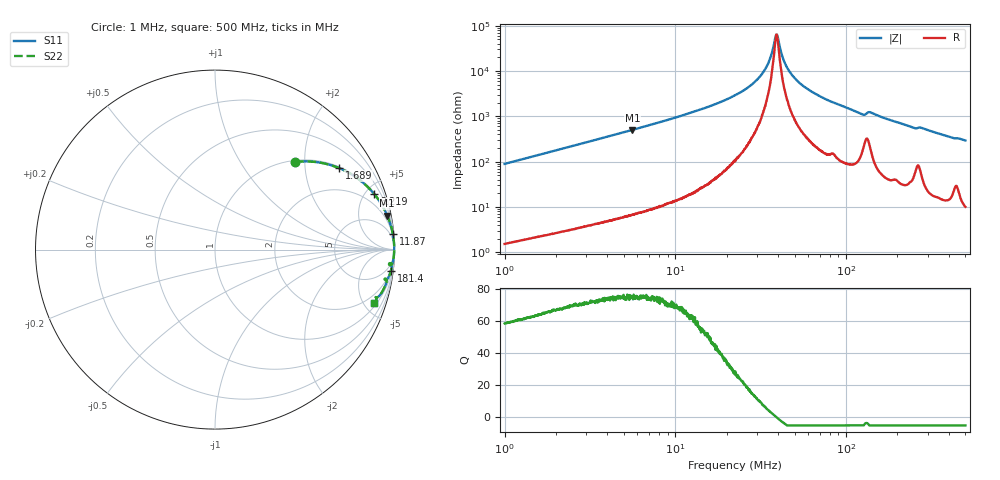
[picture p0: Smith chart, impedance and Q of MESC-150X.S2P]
!s-Parameter Generated by FASTRON Sdn. Bhd.
!FASTRON P/N : MESC-150X
!Keysight Technologies,E4991B,MY54100416,A.01.15
!Date: Mon Mar 16 10:57:22 2026
!Version  : Rev00 Mon Mar 16 10:57:22 2026
!Data & Calibration Information:
!PortZ  Port1:50+j0  Port2:50+j0
!When reading, reference impedance value at option line is always used.
!Remarks : This data is being provided solely for informational purposes.
!Freq	S11	S21	S12	S22
# Hz S dB R 50
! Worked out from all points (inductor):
!   1601 points, 1 MHz to 500 MHz, reference 50 ohm
!   read as one part in series: L = 14.2 uH near 1.032 MHz
!   highest Q = 75.5 at 5.61 MHz (marker M1), where L = 14.3 uH
!   self-resonance near 39.12 MHz
!   S11 on the Smith chart (normalised r, x): 1 MHz: 1.03, +1.79; 1.689 MHz: 1.05, +3.01; 3.219 MHz: 1.08, +5.73; 11.87 MHz: 1, +23; 181.4 MHz: 2, -17; 500 MHz: 1.20, -5.88
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1000000  -3.59 47.6  -2.63 -41.4  -2.63 -41.4  -3.59 47.6
1689373  -1.65 33.3  -5.20 -55.8  -5.20 -55.8  -1.65 33.3
2820919  -0.68 21.6  -8.67 -67.6  -8.67 -67.6  -0.68 21.6
3219169  -0.54 19.2  -9.68 -70.0  -9.68 -70.0  -0.54 19.2
5610017  -0.19 11.2  -14.25 -78.1  -14.25 -78.1  -0.19 11.2
7957584  -0.10 7.8  -17.36 -81.4  -17.36 -81.4  -0.10 7.8
1.18721e7  -0.04 5.0  -21.25 -84.1  -21.25 -84.1  -0.04 5.0
2.236068e7  -0.02 2.0  -29.31 -86.0  -29.31 -86.0  -0.02 2.0
2.779387e7  -0.01 1.2  -33.84 -85.2  -33.84 -85.2  -0.01 1.2
3.221436e7  -0.01 0.7  -38.79 -82.2  -38.79 -82.2  -0.01 0.7
3.536177e7  -0.01 0.3  -44.18 -75.9  -44.18 -75.9  -0.01 0.3
3.911941e7  -0.01 0.0  -56.19 -3.9  -56.19 -3.9  -0.01 0.0
4.004179e7  -0.01 -0.1  -54.15 37.6  -54.15 37.6  -0.01 -0.1
4.327634e7  -0.01 -0.3  -44.52 73.8  -44.52 73.8  -0.01 -0.3
4.659087e7  -0.01 -0.6  -39.85 80.0  -39.85 80.0  -0.01 -0.6
5.275702e7  -0.02 -1.0  -35.15 83.1  -35.15 83.1  -0.02 -1.0
6.307767e7  -0.02 -1.6  -30.87 84.1  -30.87 84.1  -0.02 -1.6
1.225542e8  -0.13 -5.0  -21.18 77.9  -21.18 77.9  -0.13 -5.0
1.382358e8  -0.14 -4.5  -21.97 75.9  -21.97 75.9  -0.14 -4.5
1.77937e8  -0.11 -6.7  -18.69 80.6  -18.69 80.6  -0.11 -6.7
1.814264e8  -0.11 -6.8  -18.48 80.5  -18.48 80.5  -0.11 -6.8
5e8  -0.57 -18.6  -9.93 69.5  -9.93 69.5  -0.57 -18.6
